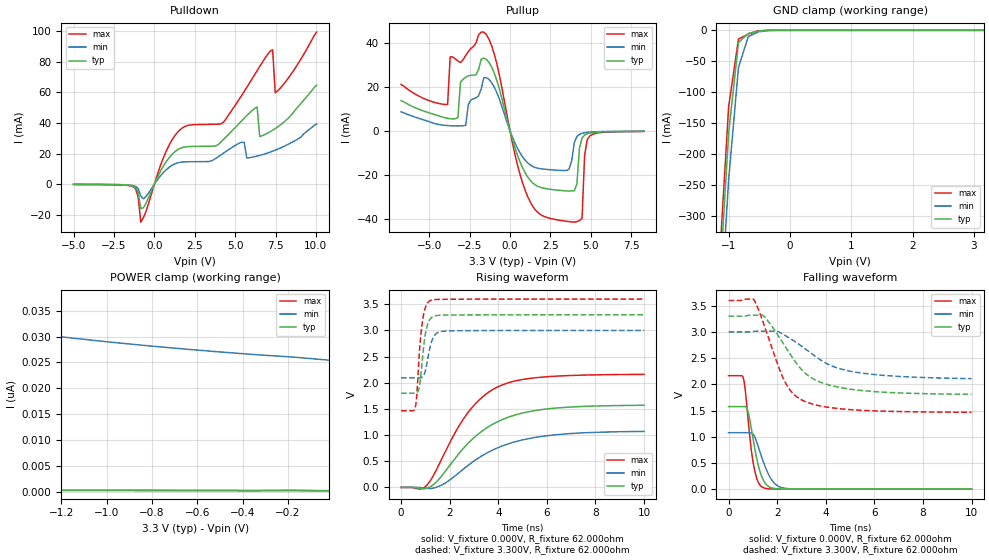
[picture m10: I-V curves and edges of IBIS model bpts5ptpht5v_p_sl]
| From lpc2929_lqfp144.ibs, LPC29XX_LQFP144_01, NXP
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| |   Rev 0.20 IBIS Model Design Automation Generation   |
| |   N O N - S I L I C O N   C O R R E L A T E D   |
| |   This IBIS [Model] is pre-Beta tactical support   |
| |  Note: this IBIS [Model] contains clamp curves generated   |
| |   through simulation which should not be relied upon   |
| Pccmos14 hliolib_nlm 4.0.1
|   0.18 um 3.3V pad library
|   six level metal
|   dual oxide
|   single threshold voltage
|   nominal line mixed supply
|   parasitic extracted netlists
| Process block c14
| bpts5ptpht5v
|   Bidirectional Pad 3v3
|   3state Output
|   Plain Input
|   1ns Slew Rate control
|   CMOS
|   Programmable between
|   - (p1=0, p2=1) plain input
|   - (p1=0, p2=0) with Pull Up
|   - (p1=1, p2=1) with Pull Down
|   - (p1=1, p2=0) with Repeater
|   Characterized at Core 1.8V and I/O 3.3V
| Plain input Mode (p1=0, p2=1)
[Model]   bpts5ptpht5v_p_sl | of bpts5ptpht5v
Model_type   I/O
Polarity   Non-Inverting
Enable   Active-Low
|  Reciever Thresholds
Vinl   = 0.99V
Vinh   = 2.31V
| AC Test Load Conditions
Vref   = 0
Cref   = 1.2e-11
Rref   = 1000000000
Vmeas   = 1.65
| [Process Range]   typical   min   max
| C_comp edge width   400.000ps   400.000ps   400.000ps
| C_comp Tstrobe   40.000fs   40.000fs   40.000fs
C_comp   2.522pF   2.389pF   2.658pF
[Temperature Range]   25   125   -40
[Voltage Range]   3.30V   3.00V   3.60V
[GND Clamp Reference]   0.00V   0.00V   0.00V
[Pulldown Reference]   0.00V   0.00V   0.00V
[POWER Clamp Reference]   3.30V   3.00V   3.60V
[Pullup Reference]   3.30V   3.00V   3.60V
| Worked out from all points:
|   slope of the pulldown table from 0 to 0.495 V, typ, clamps not added: 46.5 ohm
|   slope of the pullup table from 0 to 0.495 V, typ, clamps not added: 41.9 ohm
|   GND clamp passes 1 mA (typ) near -0.49 V on its own axis
|   rising waveform, V_fixture 0.000V, R_fixture 62.000ohm: 20-80 % time 2.15ns typ, 2.37ns min, 1.8ns max; typ from 0 V to 1.57 V
|   falling waveform, V_fixture 0.000V, R_fixture 62.000ohm: 20-80 % time 410ps typ, 536ps min, 318ps max; typ from 1.57 V to 0 V
|   rising waveform, V_fixture 3.300V, R_fixture 62.000ohm: 20-80 % time 224ps typ, 260ps min, 215ps max; typ from 1.8 V to 3.3 V
|   falling waveform, V_fixture 3.300V, R_fixture 62.000ohm: 20-80 % time 1.53ns typ, 1.95ns min, 1.09ns max; typ from 3.3 V to 1.81 V
[GND Clamp]
| ref voltage   0.00V   0.00V   0.00V
|   Voltage   I(typ)   I(min)   I(max)
-5V       -7.933A    -7.953A    -7.929A
-1.16V    -429.6mA   -501mA     -389.4mA
-1V       -166mA     -240.8mA   -123.1mA
-840mV    -19.69mA   -60.07mA   -14.09mA
-680mV    -5.152mA   -10.14mA   -6.089mA
-520mV    -1.268mA   -2.624mA   -791.9uA
-200mV    -120.2nA   -8.927uA   -2.485nA
3.16V     214.9pA    26.04nA    149.6pA
[Power Clamp]   | Vtable = Vcc - Vpad
| ref voltage   3.30V   3.00V   3.60V
|   Voltage   I(typ)   I(min)   I(max)
-6.74V    1.25nA     125.5nA    594.5pA
-4.66V    766.7pA    70.58nA    463.5pA
-2.42V    452.4pA    38.32nA    329.5pA
-2.26V    435.5pA    36.92nA    320pA
-2.1V     419.2pA    35.63nA    310.6pA
-1.78V    388.2pA    33.31nA    291.8pA
-1.62V    373.4pA    32.29nA    282.4pA
-1.3V     345pA      30.47nA    263.6pA
-980mV    318.1pA    28.92nA    244.8pA
-660mV    292.5pA    27.62nA    226.1pA
-180mV    257pA      26.06nA    260.4pA
-20mV     229.7pA    25.46nA    172.4pA
[Pulldown]
| ref voltage   0.00V   0.00V   0.00V
|   Voltage   I(typ)   I(min)   I(max)
-5V       -187.5uA   -145.7uA   -211.8uA
-1.32V    -1.32mA    -939.3uA   -1.723mA
-1V       -5.321mA   -2.96mA    -8.615mA
-840mV    -15.95mA   -7.733mA   -24.9mA
1.4V      22.26mA    13.79mA    33.48mA
4.28V     29.27mA    20.27mA    40.55mA
5.56V     43.15mA    27.33mA    60.63mA
6.36V     50.49mA    18.36mA    74.24mA
6.52V     31.16mA    18.79mA    76.97mA
7.32V     35.27mA    21.55mA    87.95mA
7.48V     36.36mA    22.22mA    59.78mA
10.04V    64.68mA    39.32mA    99.49mA
[Pullup]   | Vtable = Vcc - Vpad
| ref voltage   3.30V   3.00V   3.60V
|   Voltage   I(typ)   I(min)   I(max)
-6.74V    13.67mA    8.53mA     21.02mA
-3.86V    5.598mA    2.307mA    11.88mA
-3.7V     5.416mA    2.227mA    33.56mA
-2.74V    24.29mA    2.441mA    34.22mA
-1.62V    32.99mA    24.07mA    44.83mA
940mV     -19.18mA   -13.46mA   -27.14mA
2.86V     -27.01mA   -17.98mA   -40.52mA
3.98V     -27.38mA   -5.508mA   -41.66mA
4.46V     -3.36mA    -1.235mA   -39.9mA
4.62V     -2.02mA    -961.4uA   -11.27mA
4.94V     -1.105mA   -662.2uA   -2.417mA
8.3V      -310.5uA   -276uA     -365.2uA
[Ramp]
R_load   = 62.000ohm
|   dV/dt(typ)   dV/dt(min)   dV/dt(max)
dV/dt_r   720.645mV/2.205ns   482.706mV/2.365ns   1.049V/2.040ns
dV/dt_f   674.672mV/1.570ns   397.624mV/1.940ns   1.039V/1.250ns
[Rising Waveform]  | cubic spline decimation from 2001 points
V_fixture   = 0.000V
R_fixture   = 62.000ohm
|   Time   V(typ)   V(min)   V(max)
0s        2.056nV    364.8nV    1.069nV
765ps     -17.15mV   -3.167mV   -33.52mV
1.06ns    -16.1mV    -17.57mV   40.95mV
1.685ns   228.3mV    47.95mV    555mV
2.675ns   802.9mV    391mV      1.38V
3.325ns   1.074V     602.7mV    1.719V
3.945ns   1.249V     751mV      1.914V
4.75ns    1.392V     879.4mV    2.041V
6.04ns    1.502V     990mV      2.117V
10ns      1.57V      1.07V      2.161V
[Falling Waveform]  | cubic spline decimation from 2001 points
V_fixture   = 0.000V
R_fixture   = 62.000ohm
|   Time   V(typ)   V(min)   V(max)
0s        1.575V     1.077V     2.165V
605ps     1.575V     1.077V     2.124V
675ps     1.576V     1.076V     1.938V
790ps     1.495V     1.077V     1.404V
1.02ns    930mV      1.04V      484.7mV
1.205ns   491.3mV    835.9mV    150.3mV
1.415ns   188.7mV    541.6mV    32.06mV
1.83ns    17.74mV    142.1mV    3.549mV
2.36ns    2.451mV    14.24mV    1.422mV
10ns      41.42uV    103.1uV    18.3uV
[Rising Waveform]  | cubic spline decimation from 2001 points
V_fixture   = 3.300V
V_fixture_min = 3.000V
V_fixture_max = 3.600V
R_fixture   = 62.000ohm
|   Time   V(typ)   V(min)   V(max)
0s        1.8V       2.092V     1.464V
590ps     1.801V     2.093V     1.541V
640ps     1.808V     2.093V     1.719V
740ps     1.895V     2.092V     2.484V
870ps     2.413V     2.11V      3.136V
1.01ns    2.957V     2.248V     3.448V
1.185ns   3.209V     2.662V     3.568V
1.415ns   3.281V     2.926V     3.591V
1.77ns    3.293V     2.987V     3.596V
10ns      3.3V       3V         3.6V
[Falling Waveform]  | cubic spline decimation from 2001 points
V_fixture   = 3.300V
V_fixture_min = 3.000V
V_fixture_max = 3.600V
R_fixture   = 62.000ohm
|   Time   V(typ)   V(min)   V(max)
0s        3.3V       3V         3.6V
1.04ns    3.32V      3.009V     3.616V
1.45ns    3.304V     3.014V     3.151V
2ns       2.961V     3.01V      2.409V
2.295ns   2.749V     2.941V     2.072V
2.595ns   2.533V     2.858V     1.852V
3.055ns   2.256V     2.711V     1.692V
3.765ns   2.043V     2.471V     1.588V
5.055ns   1.904V     2.246V     1.516V
10ns      1.809V     2.109V     1.467V
